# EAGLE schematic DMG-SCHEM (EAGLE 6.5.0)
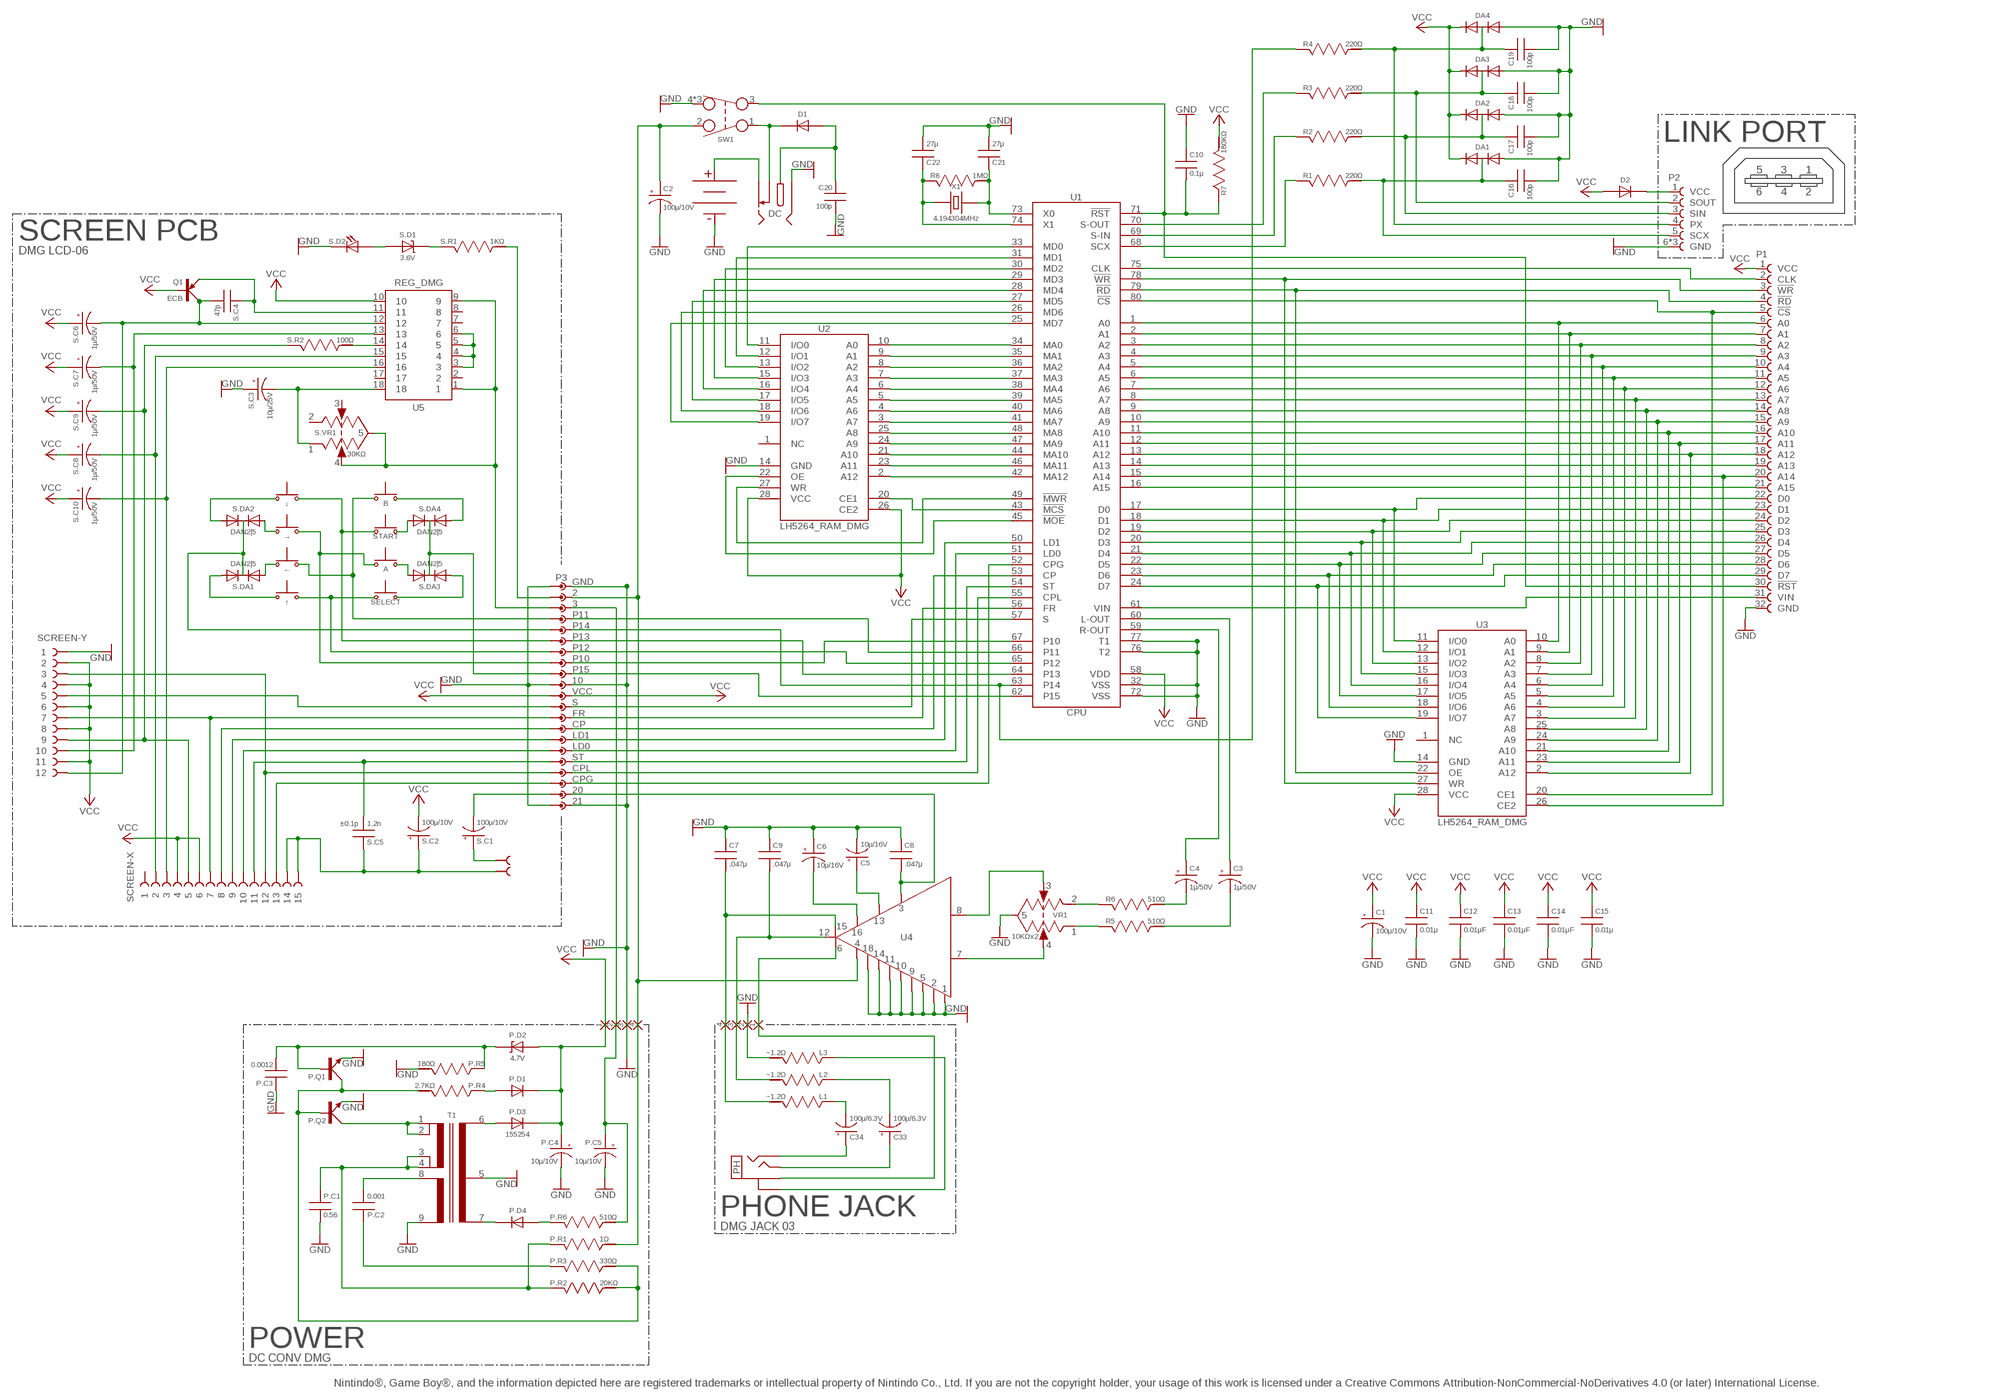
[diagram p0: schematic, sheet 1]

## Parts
A  BTN_PUSH_2_A  [DMG_BTN_A]
AUDIO  LAZY_HOLE_50MIL  [LAZY_50]
B  BTN_PUSH_2_B  [DMG_BTN_B]
C1  100μ/10V  CAPACITOR_ELECTROLYTIC_200MIL  [CAP-200E]
C2  100μ/10V  CAPACITOR_ELECTROLYTIC_200MIL  [CAP-200E]
C3  1μ/50V  CAPACITOR_ELECTROLYTIC_200MIL  [CAP-200E]
C4  1μ/50V  CAPACITOR_ELECTROLYTIC_200MIL  [CAP-200E]
C5  10μ/16V  CAPACITOR_ELECTROLYTIC_200MIL  [CAP-200E]
C6  10μ/16V  CAPACITOR_ELECTROLYTIC_200MIL  [CAP-200E]
C7  .047μ  CAPACITOR_200MIL  [CAP-200]
C8  .047μ  CAPACITOR_200MIL  [CAP-200]
C9  .047μ  CAPACITOR_200MIL  [CAP-200]
C10  0.1μ  CAPACITOR_200MIL  [CAP-200]
C11  0.01μ  CAPACITOR_200MIL  [CAP-200]
C12  0.01μF  CAPACITOR_200MIL  [CAP-200]
C13  0.01μF  CAPACITOR_200MIL  [CAP-200]
C14  0.01μF  CAPACITOR_200MIL  [CAP-200]
C15  0.01μ  CAPACITOR_200MIL  [CAP-200]
C16  100p  CAPACITOR_100MIL  [CAP-100]
C17  100p  CAPACITOR_100MIL  [CAP-100]
C18  100p  CAPACITOR_100MIL  [CAP-100]
C19  100p  CAPACITOR_100MIL  [CAP-100]
C20  100p  CAPACITOR_100MIL  [CAP-100]
C21  27μ  CAPACITOR_100MIL  [CAP-100]
C22  27μ  CAPACITOR_100MIL  [CAP-100]
C33  100μ/6.3V  CAPACITOR_ELECTROLYTIC_200MIL  [CAP-200E]
C34  100μ/6.3V  CAPACITOR_ELECTROLYTIC_200MIL  [CAP-200E]
D1  DIODE_300MIL  [DIODE-300]
D2  DIODE_300MIL  [DIODE-300]
DA1  DIODE_ARRAY_DMG  [DMG_DIODE_ARRAY@1]
DA2  DIODE_ARRAY_DMG  [DMG_DIODE_ARRAY@1]
DA3  DIODE_ARRAY_DMG  [DMG_DIODE_ARRAY@1]
DA4  DIODE_ARRAY_DMG  [DMG_DIODE_ARRAY@1]
DC  PWR_JACK_DMG  [DMG_PWR_JACK]
L1  ~1.2Ω  RESISTOR600MIL  [RES-300]
L2  ~1.2Ω  RESISTOR600MIL  [RES-300]
L3  ~1.2Ω  RESISTOR600MIL  [RES-300]
P1  DMG_SOCKET  [DMG_SOCKET]
P2  DMG_LINK_PORT  [DMG_LINK_PORT]
P3  DMG_SOCKET_SYMBOL  [DUMMY42]
P.C1  0.56  CAPACITOR_100MIL  [CAP-100]
P.C2  0.001  CAPACITOR_100MIL  [CAP-100]
P.C3  0.0012  CAPACITOR_100MIL  [CAP-100]
P.C4  10μ/10V  CAPACITOR_ELECTROLYTIC_200MIL  [CAP-200E]
P.C5  10μ/10V  CAPACITOR_ELECTROLYTIC_200MIL  [CAP-200E]
P.D1  DIODE_300MIL  [DIODE-300]
P.D2  4.7V  DIODE_ZENER  [DIODE-300]
P.D3  DIODE_300MIL  [DIODE-300]
P.D4  DIODE_300MIL  [DIODE-300]
P.Q1  TRANSISTOR_NPN  [TRANSISTOR]
P.Q2  TRANSISTOR_NPN  [TRANSISTOR]
P.R1  1Ω  RESISTOR600MIL  [RES-300]
P.R2  20KΩ  RESISTOR600MIL  [RES-300]
P.R3  330Ω  RESISTOR600MIL  [RES-300]
P.R4  2.7KΩ  RESISTOR600MIL  [RES-300]
P.R5  180Ω  RESISTOR600MIL  [RES-300]
P.R6  510Ω  RESISTOR600MIL  [RES-300]
PH  JACK_1/8"  [JACK_1/8"]
Q1  ECB  TRANSISTOR_PNP  [TRANSISTOR]
R1  220Ω  RESISTOR600MIL  [RES-300]
R2  220Ω  RESISTOR600MIL  [RES-300]
R3  220Ω  RESISTOR600MIL  [RES-300]
R4  220Ω  RESISTOR600MIL  [RES-300]
R5  510Ω  RESISTOR600MIL  [RES-300]
R6  510Ω  RESISTOR600MIL  [RES-300]
R7  180KΩ  RESISTOR600MIL  [RES-300]
R8  1MΩ  RESISTOR600MIL  [RES-300]
S.C1  100μ/10V  CAPACITOR_ELECTROLYTIC_200MIL  [CAP-200E]
S.C2  100μ/10V  CAPACITOR_ELECTROLYTIC_200MIL  [CAP-200E]
S.C3  10μ/25V  CAPACITOR_ELECTROLYTIC_200MIL  [CAP-200E]
S.C4  47p  CAPACITOR_200MIL  [CAP-200]
S.C5  1.2n  CAPACITOR_200MIL  [CAP-200]
S.C6  1μ/50V  CAPACITOR_ELECTROLYTIC_200MIL  [CAP-200E]
S.C7  1μ/50V  CAPACITOR_ELECTROLYTIC_200MIL  [CAP-200E]
S.C8  1μ/50V  CAPACITOR_ELECTROLYTIC_200MIL  [CAP-200E]
S.C9  1μ/50V  CAPACITOR_ELECTROLYTIC_200MIL  [CAP-200E]
S.C10  1μ/50V  CAPACITOR_ELECTROLYTIC_200MIL  [CAP-200E]
S.D1  3.6V  DIODE_ZENER  [DIODE-300]
S.D2  LED100MIL  [LED-100]
S.DA1  DAN2|5  DIODE_ARRAY_DMG_CENTER  [DMG_DIODE_ARRAY]
S.DA2  DAN2|5  DIODE_ARRAY_DMG_CENTER  [DMG_DIODE_ARRAY]
S.DA3  DAN2|5  DIODE_ARRAY_DMG_CENTER  [DMG_DIODE_ARRAY]
S.DA4  DAN2|5  DIODE_ARRAY_DMG_CENTER  [DMG_DIODE_ARRAY]
S.R1  1KΩ  RESISTOR600MIL  [RES-300]
S.R2  100Ω  RESISTOR600MIL  [RES-300]
S.VR1  30KΩ  POT_DMG_DMG  [DMG_POT]
SCREEN-X  CONTACT_DMG_SCREEN_X  [DMG_CONTACT_SCREEN_X]
SCREEN-Y  CONTACT_DMG_SCREEN_Y  [DMG_CONTACT_SCREEN_Y]
SELECT  BTN_PUSH_2_SELECT  [DMG_BTN_SEL]
START  BTN_PUSH_2_START  [DMG_BTN_STR]
SW1  SWITCH_DMG  [DMG_SWITCH]
T1  DMG_TRANSFORMER  [DMG_TRANSFORMER]
U1  CPU  LR35902_CPU_DMG  [LR35902_CPU_DMG]
U2  LH5264_RAM_DMG  [LH5264_RAM_DMG]
U3  LH5264_RAM_DMG  [LH5264_RAM_DMG]
U4  AMP_DMG  [AMP_DMG]
U5  REG_DMG  [REG_DMG]
U$1  LAZY_HOLE_50MIL  [LAZY_50]
U$3  4  LAZY_SOLDER_CONNECTION  [LAZY_50]
U$4  4  LAZY_SOLDER_CONNECTION  [LAZY_50]
U$5  3  LAZY_SOLDER_CONNECTION  [LAZY_50]
U$6  BAT+_DMG  [DMG_BAT+]
U$8  BAT-_DMG  [DMG_BAT-]
U$9  2  LAZY_SOLDER_CONNECTION  [LAZY_50]
U$10  1  LAZY_SOLDER_CONNECTION  [LAZY_50]
U$11  3  LAZY_SOLDER_CONNECTION  [LAZY_50]
U$12  2  LAZY_SOLDER_CONNECTION  [LAZY_50]
U$13  1  LAZY_SOLDER_CONNECTION  [LAZY_50]
VR1  10KΩx2  POT_DMG_DMG  [DMG_POT]
X1  4.194304MHz  CLOCK_DMG  [CLOCK_DMG]
←  BTN_PUSH_2_D_PAD  [DMG_BTN_D]
↑  BTN_PUSH_2_D_PAD  [DMG_BTN_D]
→  BTN_PUSH_2_D_PAD  [DMG_BTN_D]
↓  BTN_PUSH_2_D_PAD  [DMG_BTN_D]

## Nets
BAT: DC.4 U$6.POS(BAT+)
GND: C1.2(-) C2.2(-) C5.2(-) C6.1(+) C7.1 C8.1 C9.1 C10.1 C11.2 C12.2 C13.2 C14.2 C15.2 C16.2 C17.2 C18.2 C19.2 C20.2 C21.2 C22.2 DA1.1 DA2.1 DA3.1 DA4.1 DC.1 L3.2 P1.32(GND) P2.6(GND) P2.MT1(GND) P2.MT2(GND) P3.10 P3.21 P3.GND P3.P$17 P3.P$39 P3.P$41(GND) P.C1.2 P.C3.1 P.C4.2(-) P.C5.2(-) P.Q1.E P.Q2.E P.R5.2 S.C3.1(+) S.D2.1 SCREEN-Y.1 SW1.4 SW1.MT1 SW1.MT2 T1.5 T1.9 U1.32(VSS) U1.72(VSS) U1.76(T2) U1.77(T1) U2.14(GND) U3.14(GND) U4.1 U4.2 U4.5 U4.9 U4.10 U4.11 U4.14 U4.18 U$8.NEG(BAT-) U$9.X U$11.X VR1.5 VR1.MT1 VR1.MT2 ; supply symbol labelled GND_SIDE, GND_END, SUPPLY_GND_SIDE
L-OUT: C3.1(+) U1.60(L-OUT)
L-STEP1: C3.2(-) R5.2
L-STEP2: R5.1 VR1.1
L-STEP3: U4.7 VR1.4
LEFT: C7.2 L1.2 U4.15 U$4.X
N$1: P1.31(VIN) U1.61(VIN)
N$2: P3.P$3 S.VR1.4 S.VR1.5 S.VR1.MT1 S.VR1.MT2 U5.1 U5.9
N$3: D2.2 P2.1(VCC)
N$4: P1.29(D7) U1.24(D7) U3.19(I/O7)
N$5: P1.28(D6) U1.23(D6) U3.18(I/O6)
N$6: P1.27(D5) U1.22(D5) U3.17(I/O5)
N$7: P1.26(D4) U1.21(D4) U3.16(I/O4)
N$8: P1.25(D3) U1.20(D3) U3.15(I/O3)
N$9: P1.24(D2) U1.19(D2) U3.13(I/O2)
N$10: P1.23(D1) U1.18(D1) U3.12(I/O1)
N$11: P1.22(D0) U1.17(D0) U3.11(I/O0)
N$12: P1.21(A15) U1.16(A15)
N$13: P1.20(A14) U1.15(A14) U3.26(CE2)
N$14: P1.19(A13) U1.14(A13)
N$15: P1.18(A12) U1.13(A12) U3.2(A12)
N$16: P1.17(A11) U1.12(A11) U3.23(A11)
N$17: P1.16(A10) U1.11(A10) U3.21(A10)
N$18: P1.15(A9) U1.10(A9) U3.24(A9)
N$19: P1.14(A8) U1.9(A8) U3.25(A8)
N$20: P1.13(A7) U1.8(A7) U3.3(A7)
N$21: P1.12(A6) U1.7(A6) U3.4(A6)
N$22: P1.11(A5) U1.6(A5) U3.5(A5)
N$23: P1.10(A4) U1.5(A4) U3.6(A4)
N$24: P1.9(A3) U1.4(A3) U3.7(A3)
N$25: P1.8(A2) U1.3(A2) U3.8(A2)
N$26: P1.7(A1) U1.2(A1) U3.9(A1)
N$27: P1.6(A0) U1.1(A0) U3.10(A0)
N$28: P1.5(!CS) U1.80(!CS) U3.20(CE1)
N$29: P1.4(!RD) U1.79(!RD) U3.22(OE)
N$30: P1.2(CLK) U1.75(CLK)
N$31: U1.33(MD0) U2.11(I/O0)
N$32: U1.31(MD1) U2.12(I/O1)
N$33: U1.30(MD2) U2.13(I/O2)
N$34: U1.29(MD3) U2.15(I/O3)
N$35: U1.28(MD4) U2.16(I/O4)
N$36: U1.27(MD5) U2.17(I/O5)
N$37: U1.26(MD6) U2.18(I/O6)
N$38: U1.25(MD7) U2.19(I/O7)
N$39: U1.45(!MOE) U2.22(OE)
N$40: U1.49(!MWR) U2.27(WR)
N$41: U1.43(!MCS) U2.20(CE1)
N$42: U1.42(MA12) U2.2(A12)
N$43: U1.46(MA11) U2.23(A11)
N$44: U1.44(MA10) U2.21(A10)
N$45: U1.47(MA9) U2.24(A9)
N$46: U1.48(MA8) U2.25(A8)
N$47: U1.41(MA7) U2.3(A7)
N$48: U1.40(MA6) U2.4(A6)
N$49: U1.39(MA5) U2.5(A5)
N$50: U1.38(MA4) U2.6(A4)
N$51: U1.37(MA3) U2.7(A3)
N$52: U1.36(MA2) U2.8(A2)
N$53: U1.35(MA1) U2.9(A1)
N$54: U1.34(MA0) U2.10(A0)
N$55: C21.1 R8.2 U1.73(X0) X1.2
N$56: C22.1 R8.1 U1.74(X1) X1.1
N$57: P1.3(!WR) U1.78(!WR) U3.27(WR)
N$58: R3.1 U1.70(S-OUT)
N$59: R2.1 U1.69(S-IN)
N$60: P3.P$1 S.R1.2
N$61: R1.1 U1.68(SCX)
N$62: C16.1 DA1.2 P2.5(SCX) R1.2
N$63: C17.1 DA2.2 P2.3(SIN) R2.2
N$64: C18.1 DA3.2 P2.2(SOUT) R3.2
N$65: C19.1 DA4.2 P2.4(PX) R4.2
N$66: B.1 B.3 S.DA4.3
N$67: S.DA2.1 ↓.2
N$68: S.DA1.1 ←.2
N$69: S.DA1.3 ↑.1
N$70: S.DA2.3 →.1
N$71: S.DA4.1 START.2 START.3 START.6 START.7
N$72: S.DA3.1 SELECT.1 SELECT.4 SELECT.5 SELECT.8
N$73: A.2 A.4 S.DA3.3
N$74: P3.3
N$75: S.D1.2 S.R1.1
N$76: S.D1.1 S.D2.2
N$77: PH.3 U4.6 U$10.X
N$78: C6.2(-) U4.16
N$79: C8.2 P3.20 U4.3
N$80: B.2 B.4 P3.P$5 ←.1
N$81: P3.P$7 S.DA1.2 S.DA2.2
N$82: P3.P$9 START.1 START.4 START.5 START.8 ↓.1
N$83: P3.P$11 SELECT.2 SELECT.3 SELECT.6 SELECT.7 ↑.2
N$84: A.1 A.3 P3.P$13 →.2
N$85: P3.S U1.57(S)
N$86: P3.P$23 SCREEN-X.7 SCREEN-Y.7
N$87: P3.CP U1.53(CP)
N$88: P3.LD1 U1.50(LD1)
N$89: P3.LD0 U1.51(LD0)
N$90: P3.ST U1.54(ST)
N$91: P3.P$33 SCREEN-X.12 SCREEN-Y.3
N$92: P3.CPG U1.52(CPG)
N$93: P3.P$15 S.DA3.2 S.DA4.2
N$94: P3.P$21 SCREEN-Y.5
N$95: P3.FR U1.56(FR)
N$96: P3.P$25 SCREEN-X.8
N$97: P3.P$27 SCREEN-X.9
N$98: P3.P$29 SCREEN-X.10
N$99: AUDIO.X S.C1.1(+)
N$100: P3.P$31 S.C5.2 SCREEN-X.11
N$101: P3.CPL U1.55(CPL)
N$102: C5.1(+) U4.13
N$103: P3.P$35 SCREEN-X.13
N$104: U5.3 U5.4 U5.5 U5.6
N$105: P3.P$37 S.C1.2(-)
N$106: C20.1 D1.1 DC.2
N$107: S.R2.2 U5.14
N$108: Q1.E S.C4.1 U5.11
N$109: Q1.C S.C4.2 S.C6.2(-) SCREEN-Y.12 U5.12
N$110: S.C7.2(-) SCREEN-Y.10 U5.13
N$111: S.C8.2(-) SCREEN-X.2 U5.15
N$112: S.C10.2(-) SCREEN-X.3 U5.16
N$113: S.C9.2(-) S.R2.1 SCREEN-X.5 SCREEN-Y.9
N$114: S.C3.2(-) S.VR1.1 U5.18
N$115: S.C2.1(+) S.C5.1 SCREEN-X.14 SCREEN-X.15 U$1.X
N$116: P.R1.2 U$3.X
N$117: C33.1(+) PH.2
N$118: C33.2(-) L2.1
N$119: C34.2(-) L1.1
N$120: C34.1(+) PH.1
N$121: P.C1.1 P.R1.1 P.R2.1 T1.3 T1.4
N$122: P.Q2.C T1.1 T1.2
N$123: P.Q1.C P.Q2.B P.R2.2 P.R3.2 P.R4.2
N$124: L3.1 PH.G1 PH.G2
N$125: P.C2.1 P.R3.1
N$126: P.C2.2 T1.8
N$127: P.D1.1 P.R4.1
N$128: P.C3.2 P.D2.2 P.Q1.B P.R5.1
N$129: P.C4.1(+) P.D1.2 P.D2.1 P.D3.2 U$13.X
N$130: P.C5.1(+) P.R6.2 U$12.X
N$131: P.D3.1 T1.6
N$132: P.D4.1 P.R6.1
N$133: P.D4.2 T1.7
P10: P3.P10 U1.67(P10)
P11: P3.P11 U1.66(P11)
P12: P3.P12 U1.65(P12)
P13: P3.P13 U1.64(P13)
P14: P3.P14 R4.1 U1.63(P14)
P15: P3.P15 U1.62(P15)
PWR: C2.1(+) D1.2 DC.3 P3.2 SW1.1 SW1.2 U4.4
R-OUT: C4.1(+) U1.59(R-OUT)
R-STEP1: C4.2(-) R6.2
R-STEP2: R6.1 VR1.2
R-STEP3: U4.8 VR1.3
RIGHT: C9.2 L2.2 U4.12 U$5.X
RST: C10.2 P1.30(!RST) R7.1 SW1.3 U1.71(!RST)
VCC: C1.1(+) C11.1 C12.1 C13.1 C14.1 C15.1 D2.1 DA1.3 DA2.3 DA3.3 DA4.3 P1.1(VCC) P3.P$19 P3.VCC Q1.B R7.2 S.C2.2(-) S.C6.1(+) S.C7.1(+) S.C8.1(+) S.C9.1(+) S.C10.1(+) SCREEN-X.4 SCREEN-X.6 SCREEN-Y.2 SCREEN-Y.4 SCREEN-Y.6 SCREEN-Y.8 SCREEN-Y.11 U1.58(VDD) U2.26(CE2) U2.28(VCC) U3.28(VCC) U5.10 ; supply symbol labelled VCC_END, SUPPLY_VCC_END
Unconnected: S.VR1.2 S.VR1.3 SCREEN-X.1 U2.1(NC) U3.1(NC) U5.2 U5.7 U5.8 U5.17

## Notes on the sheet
- LINK PORT
- 5 | 3 | 1
- 6 | 4 | 2
- SCREEN PCB
- DMG LCD-06
- ±0.1p
- 155254
- PHONE JACK
- DMG JACK 03
- POWER
- DC CONV DMG
- Nintindo®, Game Boy®, and the information depicted here are registered trademarks or intellectual property of Nintindo Co., Ltd. If you are not the copyright holder, your usage of this work is licensed under a Creative Commons Attribution-NonCommercial-NoDerivatives 4.0 (or later) International License.

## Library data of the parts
A B SELECT START ← ↑ → ↓ = !custom:BTN_PUSH_2: Two Pin Buttons.
AUDIO U$1 = !custom:LAZY_HOLE: Connection point for something-something...
C1-C6 C33 C34 P.C4 P.C5 S.C1-S.C3 S.C6-S.C10 = !custom:CAPACITOR_ELECTROLYTIC: DMG Electrolytic Capacitor
C7-C22 P.C1-P.C3 S.C4 S.C5 = !custom:CAPACITOR: Capacitor.
D1 D2 P.D1 P.D3 P.D4 = !custom:DIODE: Diodes.
DA1-DA4 = !custom:DIODE_ARRAY_DMG: Used in DMG-01 for link-port sanitization.
DC = !custom:PWR_JACK_DMG: DC Power Jack used in DMG.
L1-L3 P.R1-P.R6 R1-R8 S.R1 S.R2 = !custom:RESISTOR: Resistor.
P1 = !custom:DMG_SOCKET: DMG Socket 32 Pin Cartridge Socket used in DMG-01
P2 = !custom:DMG_LINK_PORT: DMG Link port; used to communicate with other Gameboys.
P3 = !custom:DMG_SOCKET_SYMBOL
P.D2 S.D1 = !custom:DIODE_ZENER
P.Q1 P.Q2 = !custom:TRANSISTOR_NPN
PH = !custom:JACK_1/8"
Q1 = !custom:TRANSISTOR_PNP
S.D2 = !custom:LED: Light Emitting Diodes.
S.DA1-S.DA4 = !custom:DIODE_ARRAY_DMG_CENTER
S.VR1 VR1 = !custom:POT_DMG: Volume/Contrast Potentiomentor used on DMG-01. Based off a common thumb-wheel potentiometer that matches board.
SCREEN-X = !custom:CONTACT_DMG_SCREEN_X
SCREEN-Y = !custom:CONTACT_DMG_SCREEN_Y
SW1 = !custom:SWITCH_DMG: Power switch used in DMG.
T1 = !custom:DMG_TRANSFORMER
U1 = !custom:LR35902_CPU: Sharp LR35902 CPU Z80/8080 Hybrid used in the DMG-01 The origional spec cannot be found, so assumptions are made. This thin quad flat pack (TQFP) uses a common spacing of 0.8mm between the pins. When compaired to a scaled photo, the solder pads match very closely.
U2 U3 = !custom:LH5264_RAM: LH5264 RAM Memory used in DMG-01 Original spec sheet cannot be found. This part is based off a currently used SHARP 28SOP footprint (SOP025-P-0450). When compared to scaled photo of DMG pads, this footprint's center of tolerance matches perfectly. Pads extended to 2mm.
U4 = !custom:AMP_DMG: Gameboy Audio Amp. There is no information on this that can be found. All measurements were taken with a caliper with a resolution of 0.01mm/.5mil. Measurements were attempted in both mm and mil. The closest round number was chosen for every dimension, then re-measured for accuracy.
U5 = !custom:REG_DMG
U$3-U$5 U$9-U$13 = !custom:LAZY_SOLDER_CONNECTION
U$6 = !custom:BAT+_DMG: Positive battery contact for DMG.
U$8 = !custom:BAT-_DMG: Negative battery contact for DMG.
X1 = !custom:CLOCK: Crystal Oscillator.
